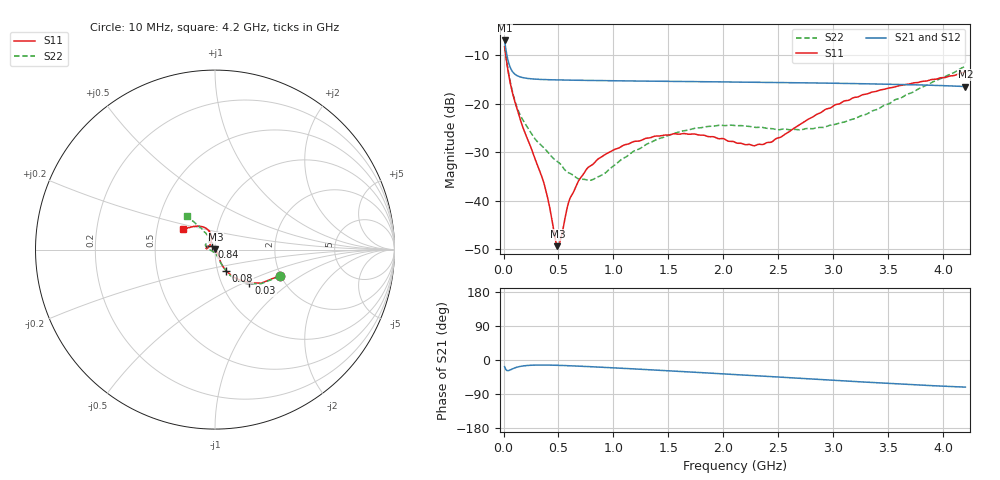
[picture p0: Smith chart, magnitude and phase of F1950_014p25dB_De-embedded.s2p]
! Integrated Device Technology
! Corporate Headquarters
! 6024 Silver Creek Valley Road
! San Jose, CA 95138  USA
! Phone:  1-408-284-8200
! Toll Free:  1-800-223-1366
! Webpage:  http://www.idt.com/
! Timing and RF Division
! 515 Groton Road, Suite 102
! Westford, MA 01886-6024
! Device:  F1950
! Description: 7-bit 0.25 dB Digital Step Attenuator
! Frequency:  150.0 -  4000.00 MHz
! Package:  4x4 mm Thin QFN Plastic Package: 24 pin
! Ports:  2 RF, 12 DC
!  Pin  1  = D0
!  Pin  2  = VDD
!  Pin  3  = Vmode
!  Pin  4  = GND
!  Pin  5  = RF1  =  Port 1
!  Pin  6  = GND
!  Pin  7  = GND
!  Pin  8  = GND
!  Pin  9  = GND
!  Pin 10  = GND
!  Pin 11  = GND
!  Pin 12  = GND
!  Pin 13  = GND
!  Pin 14  = RF2  =  Port 2
!  Pin 15  = GND
!  Pin 16  = LE
!  Pin 17  = CLK
!  Pin 18  = DATE
!  Pin 19  = D6
!  Pin 20  = D5
!  Pin 21  = D4
!  Pin 22  = D3
!  Pin 23  = D2
!  Pin 24  = D1
! State:  57
! Atten State:  14.25 dB
! Voltage:  +5.00 Volts
! Current:  Not Measured mA
! Data:  The device was measured on a the F195X evaluation board which has
!  individual transmission lines to the RF pins.  Data was collected
!  using a calibrated network analyzer.  The evaluation board was
!  de-embedded using a TRL calibration technique.
!  The reference plane is the edge of the package pin.
! Misc:  Board 2019
!  Action Tracker AT0250
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# GHz S dB R 50
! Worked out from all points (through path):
!   420 points, 10 MHz to 4.2 GHz, reference 50 ohm
!   highest |S21| = -6.94 dB at 10 MHz (marker M1); lowest = -16.5 dB at 4.2 GHz (marker M2)
!   group delay of S21, straight-line fit = 41.6 ps
!   lowest |S11| = -49.4 dB at 490 MHz (marker M3), VSWR 1.01, Z = 50.3 + j0.209 ohm
!   |S11| at or under -10 dB: 20.41 MHz to end of sweep
!   |S22| runs from -35.8 to -8.2 dB; largest |S21 - S12| = 0.00025
!   S11 on the Smith chart (normalised r, x): 10 MHz: 1.97, -0.68; 30 MHz: 1.34, -0.54; 80 MHz: 1.10, -0.26; 840 MHz: 0.96, +0.03; 4.2 GHz: 0.68, +0.16
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0.01  -8.22 -22.0  -6.94 -17.6  -6.94 -17.6  -8.19 -22.5
0.03  -11.55 -44.4  -9.88 -27.7  -9.88 -27.7  -11.44 -45.3
0.08  -17.61 -62.3  -13.31 -23.6  -13.31 -23.6  -17.39 -62.4
0.17  -24.46 -64.3  -14.58 -16.0  -14.58 -16.0  -23.12 -68.6
0.36  -35.86 -47.7  -15.00 -13.3  -15.00 -13.3  -28.94 -73.4
0.41  -40.33 -39.1  -15.04 -13.4  -15.04 -13.4  -30.18 -74.0
0.47  -47.81 3.3  -15.07 -13.8  -15.07 -13.8  -31.58 -80.3
0.49  -49.38 37.7  -15.08 -14.0  -15.08 -14.0  -31.91 -82.0
0.52  -47.90 79.2  -15.10 -14.3  -15.10 -14.3  -32.51 -83.2
0.6  -39.77 116.1  -15.13 -15.1  -15.13 -15.1  -34.33 -95.1
0.71  -35.03 128.4  -15.16 -16.5  -15.16 -16.5  -35.58 -114.1
0.84  -31.85 137.0  -15.20 -18.3  -15.20 -18.3  -35.31 -142.0
1.1  -28.48 152.7  -15.28 -22.2  -15.28 -22.2  -31.13 -176.7
1.41  -26.65 166.0  -15.36 -27.0  -15.36 -27.0  -27.22 168.3
1.73  -26.23 173.3  -15.43 -32.2  -15.43 -32.2  -25.11 159.2
2.11  -28.00 164.0  -15.52 -38.5  -15.52 -38.6  -24.52 149.7
2.28  -28.67 146.7  -15.57 -41.3  -15.56 -41.4  -24.83 144.6
2.43  -27.95 129.1  -15.60 -43.7  -15.60 -43.8  -25.10 139.8
2.81  -22.75 105.9  -15.71 -50.2  -15.70 -50.3  -25.14 124.4
3.1  -19.41 107.8  -15.80 -55.2  -15.80 -55.2  -23.76 118.9
3.51  -16.72 118.8  -15.97 -61.8  -15.96 -61.9  -19.94 119.2
4.2  -13.44 147.7  -16.45 -71.5  -16.45 -71.6  -12.26 130.0
